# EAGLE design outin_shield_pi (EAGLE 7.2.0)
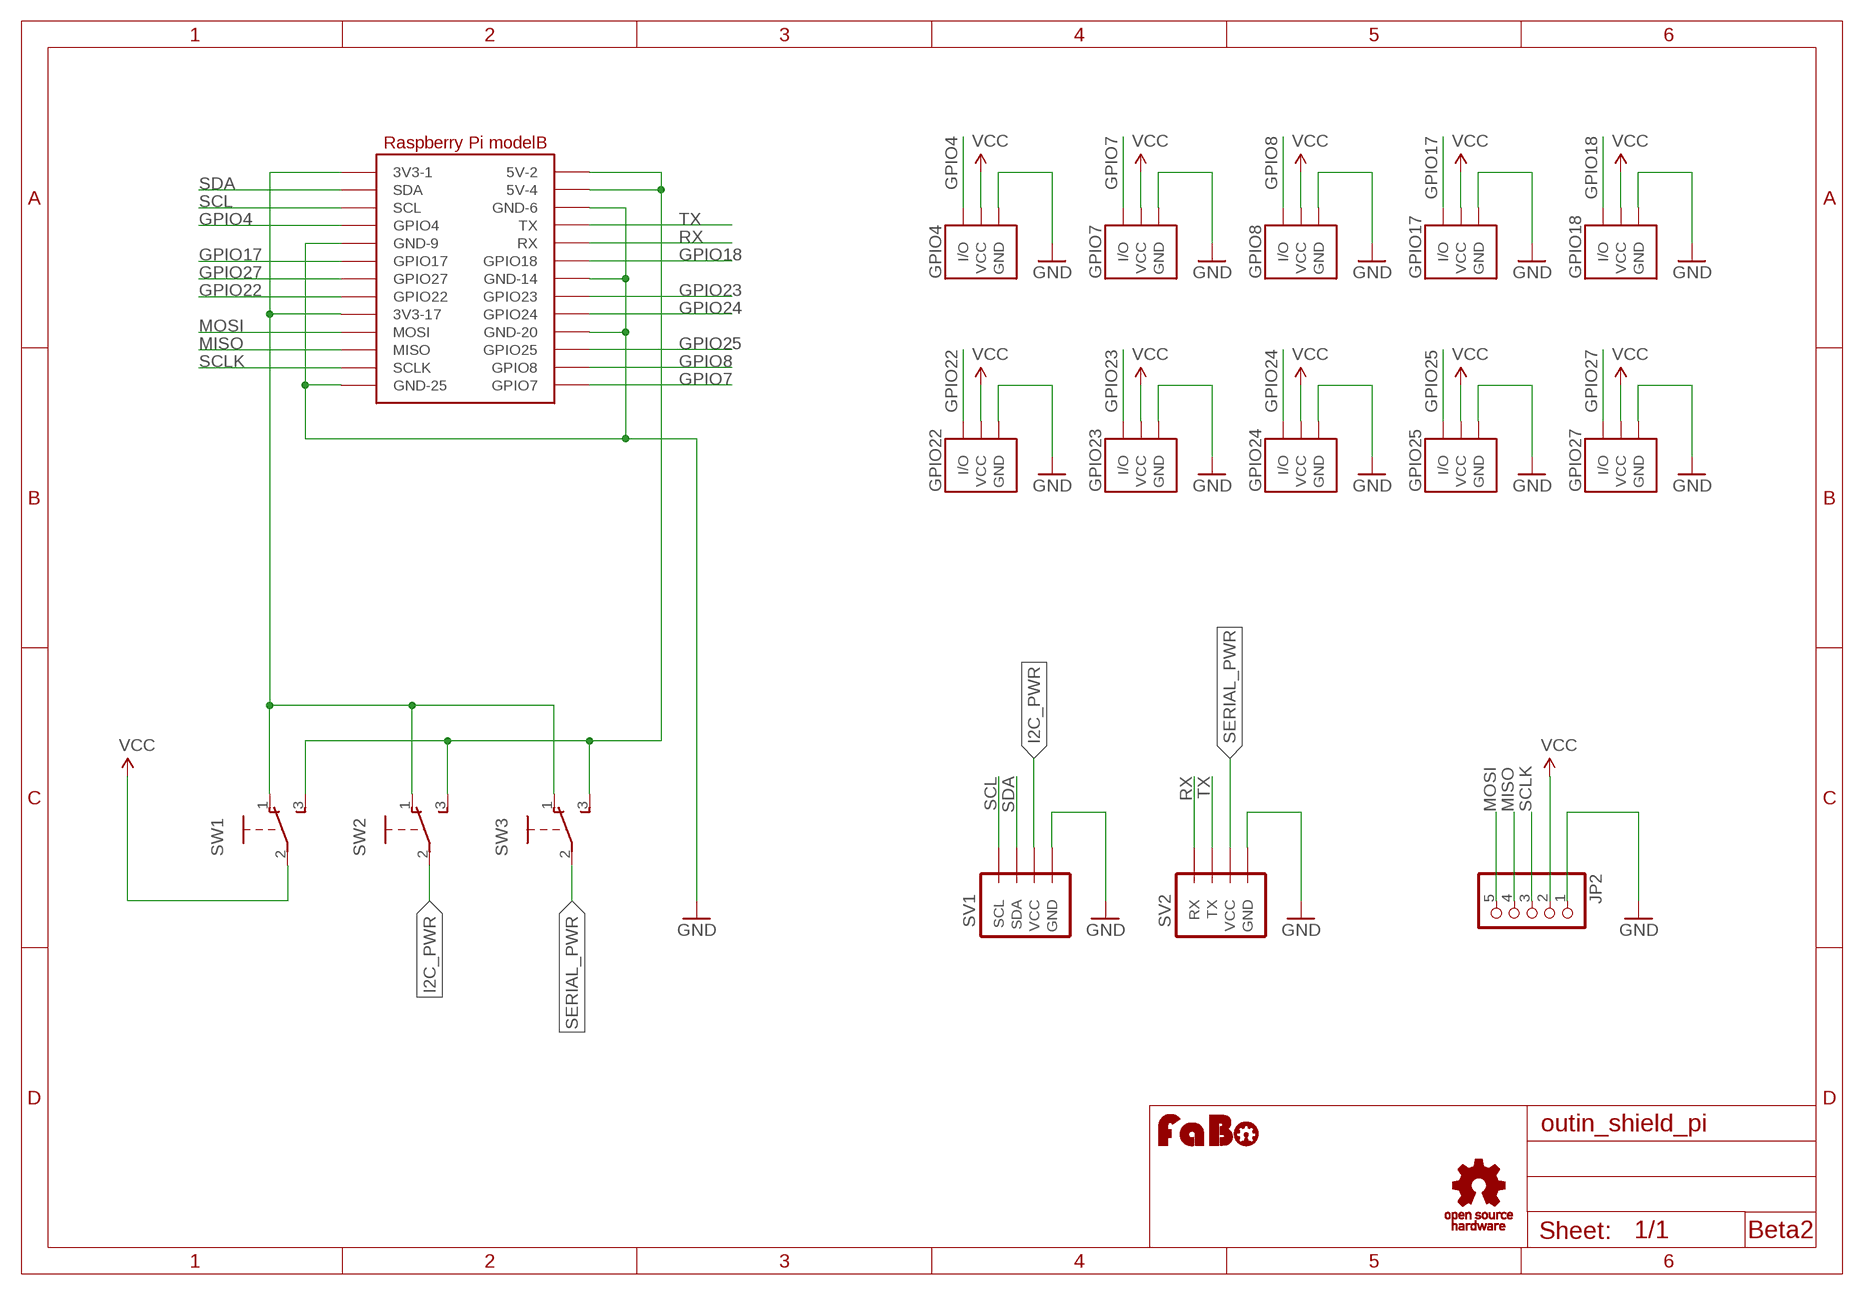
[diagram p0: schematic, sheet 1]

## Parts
GPIO4  IO_PIN-3PIN  [1X3-SNEAKY]
GPIO7  IO_PIN-3PIN  [1X3-SNEAKY]
GPIO8  IO_PIN-3PIN  [1X3-SNEAKY]
GPIO17  IO_PIN-3PIN  [1X3-SNEAKY]
GPIO18  IO_PIN-3PIN  [1X3-SNEAKY]
GPIO22  IO_PIN-3PIN  [1X3-SNEAKY]
GPIO23  IO_PIN-3PIN  [1X3-SNEAKY]
GPIO24  IO_PIN-3PIN  [1X3-SNEAKY]
GPIO25  IO_PIN-3PIN  [1X3-SNEAKY]
GPIO27  IO_PIN-3PIN  [1X3-SNEAKY]
JP2  PINHD-1X5  [1X05]
SV1  BRICK_I2C_CONNECTOR  [BRICK_I2C_CONNECTOR]
SV2  BRICK_SERIAL_CONNECTOR  [BRICK_SERIAL_CONNECTOR]
SW1  SWITCH-SLIDE-EG1218  [EG1218]
SW2  SWITCH-SLIDE-EG1218  [EG1218]
SW3  SWITCH-SLIDE-EG1218  [EG1218]
U1  RASPBERRY_PI_B1  [RASPBERRY_PI_B]
U$14  LOGO_FABO-M  [LOGO_FABO_M]
U$15  LOGO_OSHW_T-M  [LOGO_OSHW_T_M]

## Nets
3V3: SW1.1 SW2.1 SW3.1 U1.1(3V3-1) U1.17(3V3-17)
5V: SW1.3 SW2.3 SW3.3 U1.2(5V-2) U1.4(5V-4)
GND: GPIO4.1(GND) GPIO7.1(GND) GPIO8.1(GND) GPIO17.1(GND) GPIO18.1(GND) GPIO22.1(GND) GPIO23.1(GND) GPIO24.1(GND) GPIO25.1(GND) GPIO27.1(GND) JP2.1 SV1.GND SV2.GND U1.6(GND-6) U1.9(GND-9) U1.14(GND-14) U1.20(GND-20) U1.25(GND-25)
GPIO4: GPIO4.3(I/O) U1.7(GPIO4)
GPIO7: GPIO7.3(I/O) U1.26(GPIO7)
GPIO8: GPIO8.3(I/O) U1.24(GPIO8)
GPIO17: GPIO17.3(I/O) U1.11(GPIO17)
GPIO18: GPIO18.3(I/O) U1.12(GPIO18)
GPIO22: GPIO22.3(I/O) U1.15(GPIO22)
GPIO23: GPIO23.3(I/O) U1.16(GPIO23)
GPIO24: GPIO24.3(I/O) U1.18(GPIO24)
GPIO25: GPIO25.3(I/O) U1.22(GPIO25)
GPIO27: GPIO27.3(I/O) U1.13(GPIO27)
I2C_PWR: SV1.VCC SW2.2
MISO: JP2.4 U1.21(MISO)
MOSI: JP2.5 U1.19(MOSI)
RX: SV2.RX U1.10(RX)
SCL: SV1.SCL U1.5(SCL)
SCLK: JP2.3 U1.23(SCLK)
SDA: SV1.SDA U1.3(SDA)
SERIAL_PWR: SV2.VCC SW3.2
TX: SV2.TX U1.8(TX)
VCC: GPIO4.2(VCC) GPIO7.2(VCC) GPIO8.2(VCC) GPIO17.2(VCC) GPIO18.2(VCC) GPIO22.2(VCC) GPIO23.2(VCC) GPIO24.2(VCC) GPIO25.2(VCC) GPIO27.2(VCC) JP2.2 SW1.2

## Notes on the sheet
- Beta2

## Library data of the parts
GPIO4 GPIO7 GPIO8 GPIO17 GPIO18 GPIO22-GPIO25 GPIO27 = Gclue:IO_PIN
JP2 = pinhead:PINHD-1X5: PIN HEADER
SV1 = Gclue:BRICK_I2C_CONNECTOR: Brick Connector female for OUT/IN Shield
SV2 = Gclue:BRICK_SERIAL_CONNECTOR
SW1-SW3 = Gclue:SWITCH-SLIDE
U1 = Gclue:RASPBERRY_PI_B
U$14 = FaBo:LOGO_FABO
U$15 = Gclue:LOGO_OSHW_T

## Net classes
0 default: width 0.254 mm

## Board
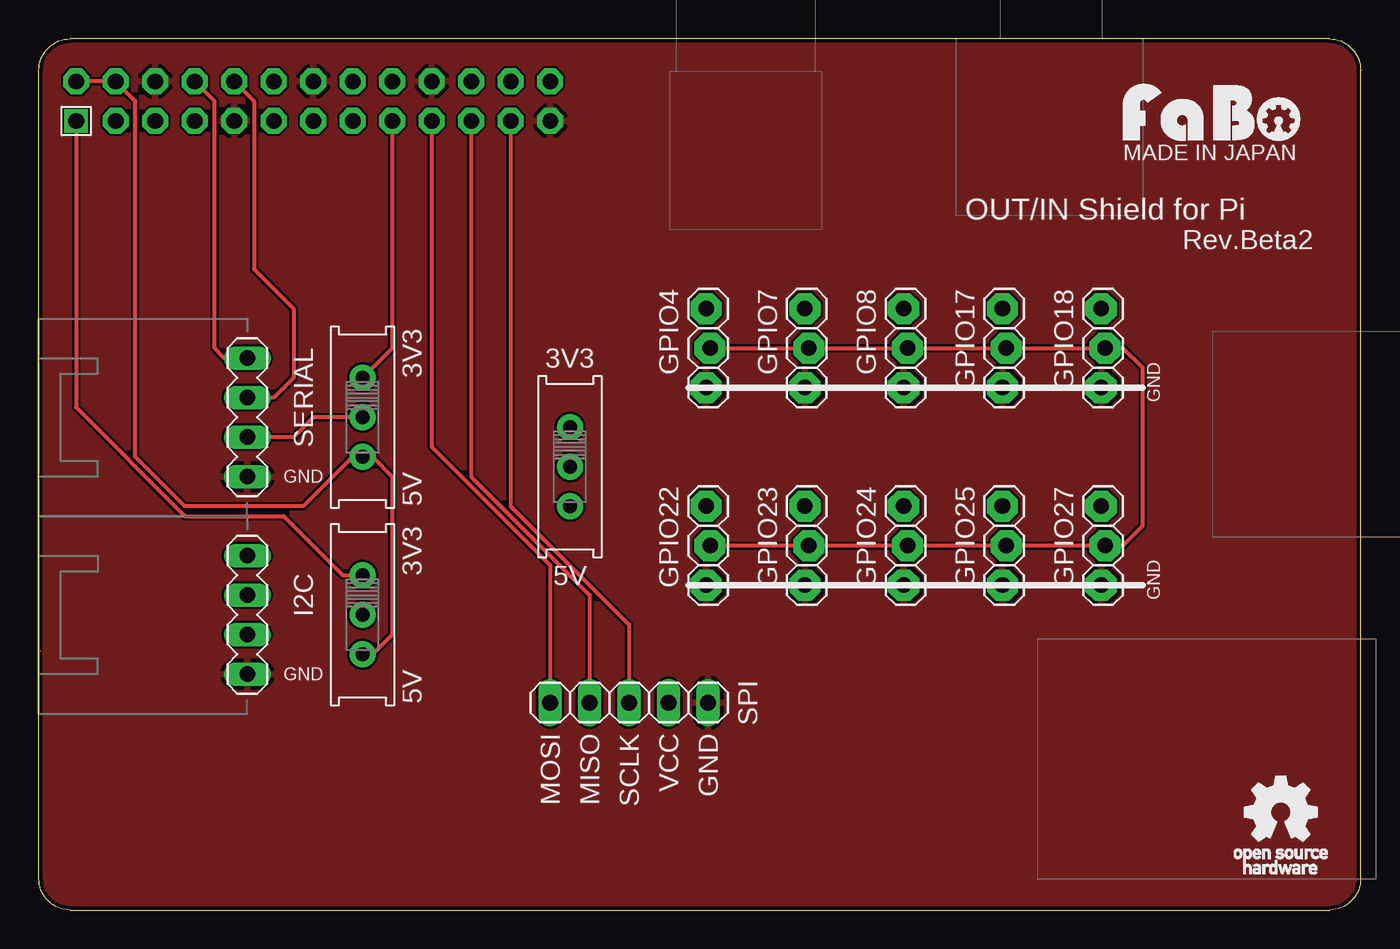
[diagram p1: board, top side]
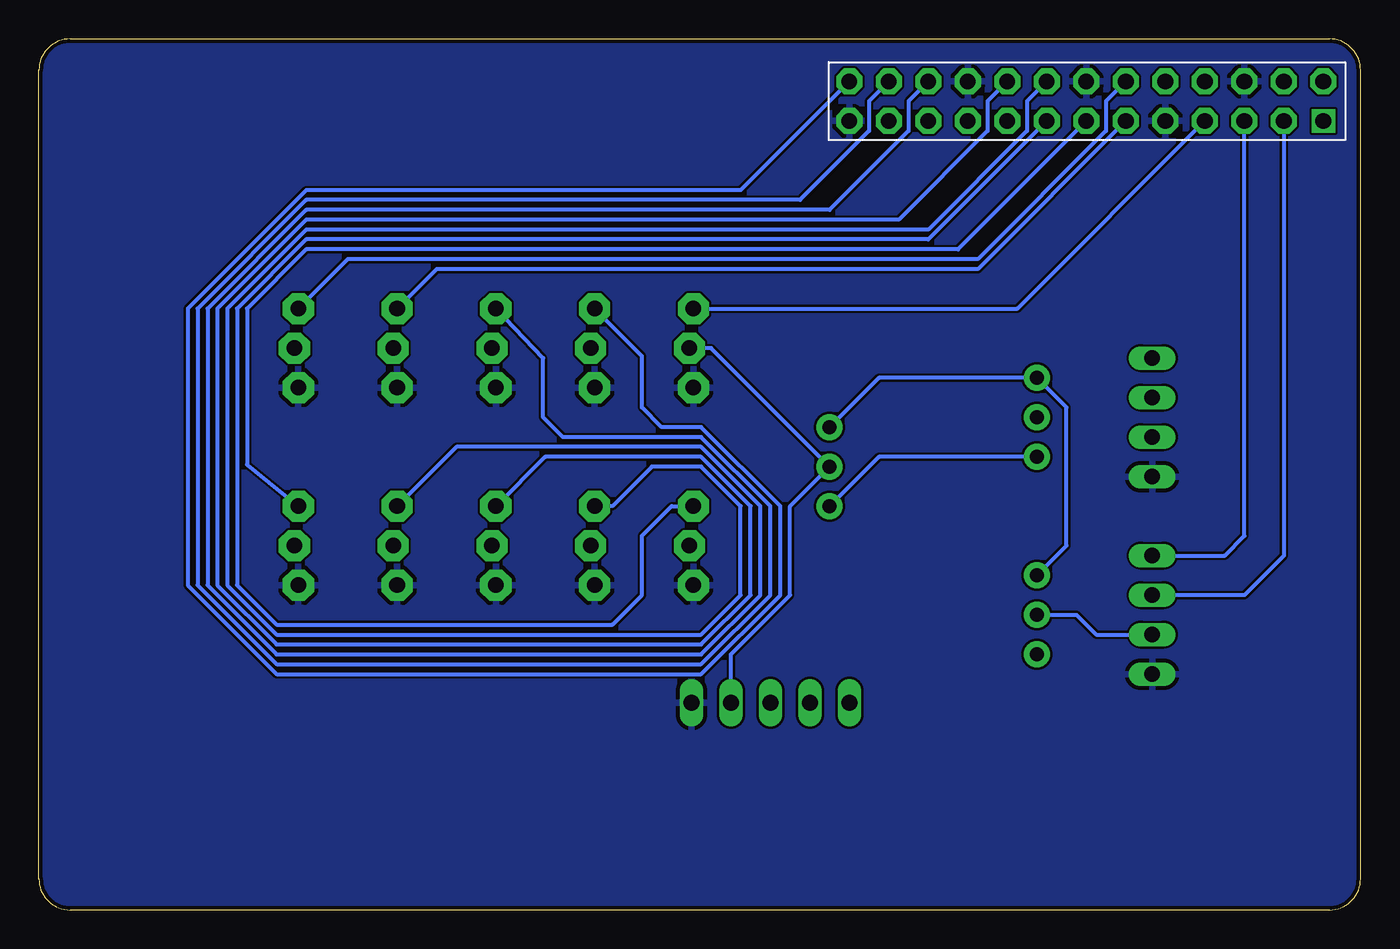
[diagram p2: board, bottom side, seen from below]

Size 85 x 56 mm. Coordinates in mm from the lower left corner, seen from the top.
Copper layers (1*16): Top 0.035mm / dielectric 1.5mm / Bottom 0.035mm
Design rules "Elecrow_2-layer_eagle_rule": minimum track width 6mil, minimum drill 12mil, track to track 6mil, track to pad 6mil, pad to pad 6mil, via to via 6mil, smd to smd 0mil, copper to edge 10mil, drill to drill 10mil, minimum pad ring 10mil, minimum via ring 6mil, stop-mask expansion 2mil, vias tented up to drill 100mil, thermal gap 10mil

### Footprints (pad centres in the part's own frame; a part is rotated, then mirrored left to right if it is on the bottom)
1X3-SNEAKY = drill 1 pad 2 octagon: 1 -2.54,0.127; 2 0,-0.127; 3 2.54,0.127
1X05 = drill 1.016 long: 1 -5.08,0; 2 -2.54,0; 3 0,0; 4 2.54,0; 5 5.08,0
BRICK_I2C_CONNECTOR = drill 1 long: GND -3.81,0; SCL 3.81,0; SDA 1.27,0; VCC -1.27,0
BRICK_SERIAL_CONNECTOR = drill 1 long: GND -3.81,0; RX 1.27,0; TX 3.81,0; VCC -1.27,0
EG1218 = drill 0.9 pad 1.676: 1 -2.54,0; 2 0,0; 3 2.54,0
RASPBERRY_PI_B = drill 1 square: 1 2.54,50.8 | drill 1 pad 1.676 octagon: 2 2.54,53.34; 3 5.08,50.8; 4 5.08,53.34; 5 7.62,50.8; 6 7.62,53.34; 7 10.16,50.8; 8 10.16,53.34; 9 12.7,50.8; 10 12.7,53.34; 11 15.24,50.8; 12 15.24,53.34; 13 17.78,50.8; 14 17.78,53.34; 15 20.32,50.8; 16 20.32,53.34; 17 22.86,50.8; 18 22.86,53.34; 19 25.4,50.8; 20 25.4,53.34; 21 27.94,50.8; 22 27.94,53.34; 23 30.48,50.8; 24 30.48,53.34; 25 33.02,50.8; 26 33.02,53.34

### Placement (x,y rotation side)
GPIO4  43.04,36.12 90 top
GPIO7  49.39,36.12 90 top
GPIO8  55.74,36.12 90 top
GPIO17  62.09,36.12 90 top
GPIO18  68.44,36.12 90 top
GPIO22  43.04,23.42 90 top
GPIO23  49.39,23.42 90 top
GPIO24  55.74,23.42 90 top
GPIO25  62.09,23.42 90 top
GPIO27  68.44,23.42 90 top
JP2  37.96,13.33 180 top
SV1  13.4,18.98 90 top
SV2  13.4,31.68 90 top
SW1  34.15,28.5 270 top
SW2  20.81,18.98 270 top
SW3  20.81,31.68 270 top
U1  -0.14,-0.07 0 top
U$14  75.42,49.45 0 top
U$15  79.87,6.27 0 top

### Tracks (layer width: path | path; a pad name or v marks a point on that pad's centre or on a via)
3V3
  Top 0.254: U1.1 2.4,32.31 9.38,25.32 15.73,25.32 19.54,21.52 SW2.1 | U1.17 22.72,36.12 SW3.1
  Bottom 0.254: SW1.1 30.97,34.21 SW3.1 18.91,32.31 18.91,23.42 SW2.1
5V
  Top 0.254: U1.2 U1.4 6.21,51.99 6.21,29.14 9.38,25.96 17,25.96 20.18,29.14 SW3.3 21.45,29.14 22.72,27.87 22.72,17.71 21.45,16.44 SW2.3
  Bottom 0.254: SW3.3 30.97,29.14 SW1.3
GND
  pour Bottom: -1.41,-1.34 86.22,-1.34 86.22,57.07 -1.41,57.07
  pour Top: -1.41,-1.34 86.22,-1.34 86.22,57.07 -1.41,57.07
GPIO4
  Bottom 0.254: GPIO4.3 22.09,38.66 U1.7
GPIO7
  Bottom 0.254: U1.26 39.87,46.28 67.8,46.28 75.42,38.66 75.42,20.88 69.71,15.17 42.41,15.17 37.33,20.25 37.33,25.96 42.41,31.04 44.95,31.04 46.21,32.31 46.21,35.61 GPIO7.3
GPIO8
  Bottom 0.254: U1.24 31.61,51.99 31.61,50.09 36.05,45.64 67.8,45.64 74.79,38.66 74.79,20.88 69.71,15.8 42.41,15.8 37.96,20.25 37.96,25.96 42.41,30.41 51.3,30.41 52.56,31.68 52.56,35.48 GPIO8.3
GPIO17
  Bottom 0.254: U1.11 24.62,41.2 59.42,41.2 GPIO17.3
GPIO18
  Bottom 0.254: U1.12 16.37,51.99 16.37,50.09 24.62,41.83 65.14,41.83 GPIO18.3
GPIO22
  Bottom 0.254: U1.15 27.8,43.1 67.8,43.1 72.25,38.66 72.25,20.88 69.71,18.34 48.12,18.34 46.21,20.25 46.21,24.05 44.31,25.96 GPIO22.3
GPIO23
  Bottom 0.254: U1.16 21.45,51.99 21.45,50.09 27.8,43.74 67.8,43.74 72.89,38.66 72.89,20.88 69.71,17.71 42.41,17.71 39.87,20.25 39.87,25.96 42.41,28.5 45.58,28.5 48.12,25.96 GPIO23.3
GPIO24
  Bottom 0.254: U1.18 23.99,51.99 23.99,50.09 29.7,44.38 67.8,44.38 73.52,38.66 73.52,20.88 69.71,17.07 42.41,17.07 39.23,20.25 39.23,25.96 42.41,29.14 52.44,29.14 GPIO24.3
GPIO25
  Bottom 0.254: U1.22 29.07,51.99 29.07,50.09 34.15,45.01 67.8,45.01 74.16,38.66 74.16,20.88 69.71,16.44 42.41,16.44 38.59,20.25 38.59,25.96 42.41,29.77 58.15,29.77 GPIO25.3
GPIO27
  Bottom 0.254: U1.13 25.89,42.47 67.8,42.47 71.61,38.66 71.61,28.63 GPIO27.3
I2C_PWR
  Bottom 0.254: SW2.2 18.27,18.98 17,17.71 SV1.VCC
MISO
  Top 0.254: U1.21 27.8,27.87 35.42,20.25 JP2.4
MOSI
  Top 0.254: U1.19 25.26,29.77 32.88,22.15 JP2.5
RX
  Top 0.254: U1.10 13.83,51.99 13.83,41.2 16.37,38.66 16.37,34.21 15.1,32.95 SV2.RX
SCL
  Bottom 0.254: SV1.SCL 8.75,22.79 7.48,24.05 U1.5
SCLK
  Top 0.254: U1.23 30.34,25.96 37.96,18.34 JP2.3
SDA
  Bottom 0.254: U1.3 4.94,22.79 7.48,20.25 SV1.SDA
SERIAL_PWR
  Top 0.254: SW3.2 17.64,31.68 16.37,30.41 SV2.VCC
TX
  Top 0.254: SV2.TX 11.92,35.48 11.29,36.12 11.29,51.99 U1.8
VCC
  Top 0.254: GPIO22.2 GPIO23.2 GPIO24.2 GPIO25.2 GPIO27.2 69.71,23.42 70.98,24.69 70.98,34.85 69.71,36.12 GPIO18.2 GPIO17.2 GPIO8.2 GPIO7.2 GPIO4.2
  Bottom 0.254: GPIO4.2 41.77,36.12 SW1.2 36.69,25.96 36.69,20.25 40.5,16.44 JP2.2

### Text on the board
tPlace: MADE IN JAPAN | OUT/IN Shield for Pi | Rev.Beta2 | 3V3 | 3V3 | SERIAL | GND | GND | 5V | 3V3 | 5V | I2C | GND | GND | 5V | SPI | MOSI | MISO | SCLK | VCC | GND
